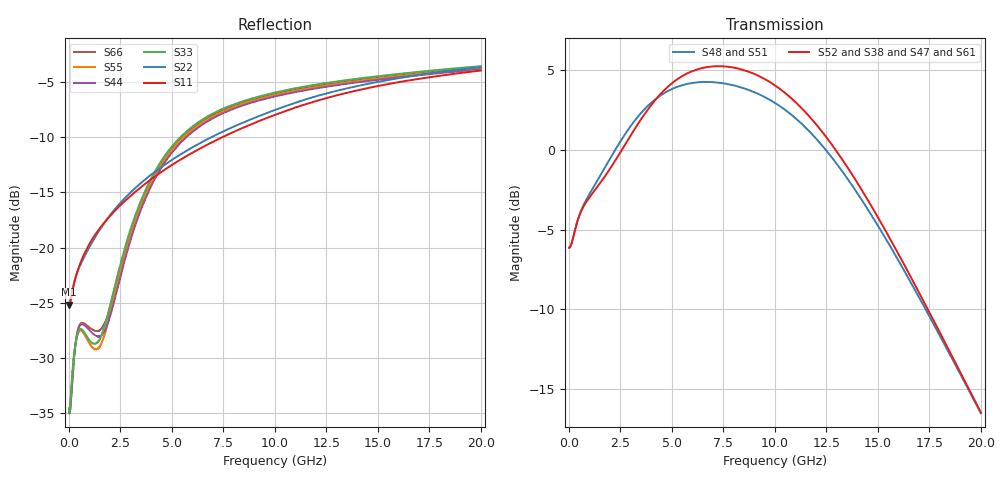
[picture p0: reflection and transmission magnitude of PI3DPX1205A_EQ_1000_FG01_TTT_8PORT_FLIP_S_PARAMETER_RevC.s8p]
! NPort=8 DATA=2000 NOISE=0 GROUPDELAY=0 COMPLEX_DATAFORMAT=POLAR
! NumOfBlock=1 NumOfParam=0
! .MODEL Smodel S TSTONEFILE=PI3DPX1205A_EQ_1000_FG01_TTT_8PORT_FLIP_S_PARAMETER_RevC.s8p TYPE=S
!  -- The above .MODEL line can be used for the S element in the netlist.
! The s parameter is extracted from the linear redriver, it is not bi-directional;
! only s(5,1)s(6,2)s(3,7)s(4,8) should be the insertion loss
!  Port definition:
!  Port1 = AIP
!  Port2 = AIN
!  Port3 = BOP
!  Port4 = BON
!  Port5 = AOP
!  Port6 = AON
!  Port7 = BIP
!  Port8 = BIN
# Hz S MA R  50
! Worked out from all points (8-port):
!   2000 points, 10 MHz to 20 GHz, reference 50 ohm
!   strongest paths, dB at 10 MHz, 5.01 GHz, 10.01 GHz, 15.01 GHz, 20 GHz:
!     S52: -6.1, 4.2, 4.0, -4.3, -16.5
!     S38: -6.1, 4.2, 4.0, -4.3, -16.5
!     S47: -6.1, 4.2, 4.1, -4.2, -16.4
!     S61: -6.1, 4.2, 4.0, -4.2, -16.4
!     S48: -6.1, 3.8, 2.9, -4.8, -16.5
!     S51: -6.1, 3.8, 2.9, -4.8, -16.5
!   lowest |S11| = -25.2 dB at 10 MHz (marker M1), VSWR 1.12, Z = 44.8 - j0.115 ohm
!   |S11| at or under -10 dB: start of sweep to 7.461 GHz
